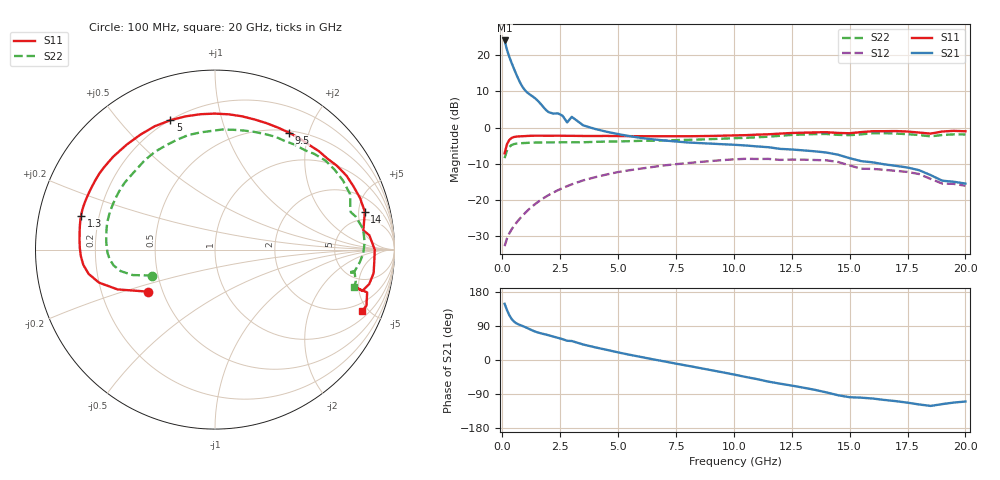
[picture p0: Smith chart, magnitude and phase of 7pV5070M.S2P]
! Infineon Technologies  Discrete & RF Semiconductors
! bfp620
! VCE = 0.50 V,  IC =  70 mA
! Common Emitter S-Parameters:  Sep 2002
# GHz  S  MA  R  50
!  f  S11  S21  S12  S22
! GHz  MAG  ANG  MAG  ANG  MAG  ANG  MAG  ANG
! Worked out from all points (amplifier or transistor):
!   59 points, 100 MHz to 20 GHz, reference 50 ohm
!   highest |S21| = 24.1 dB at 100 MHz (marker M1)
!   |S21| within 3 dB of that: start of sweep to 223.3 MHz
!   unconditionally stable (mu >= 1): start of sweep to 273.5 MHz; 598.9 MHz to 13.05 GHz; 14.34 GHz to end of sweep
!   at 1 GHz: K = 1.13, MAG = 14.6 dB, |S12| = -23.5 dB
!   at 5.5 GHz: K = 1.21, MAG = 1.9 dB, |S12| = -11.8 dB
!   at 20 GHz: K = 2.15, MAG = -5.8 dB, |S12| = -16.1 dB
!   S11 on the Smith chart (normalised r, x): 100 MHz: 0.42, -0.24; 1.3 GHz: 0.13, +0.12; 5 GHz: 0.20, +0.69; 9.5 GHz: 0.53, +1.69; 14 GHz: 3.60, +5.87; 20 GHz: 1.42, -4.56
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0.1  0.4389 -147.7  15.98 148.4  0.0229 27.2  0.3771 -157.5
0.2  0.5868 -157.8  11.93 132.1  0.0291 33.1  0.4798 -162.8
0.3  0.6719 -164.1  9.518 118.5  0.0343 37.2  0.5395 -167.2
0.4  0.7169 -169.1  7.853 108.5  0.039 40.5  0.5724 -171.2
0.5  0.7387 -173.4  6.545 101.6  0.0435 43.1  0.5898 -174.9
0.6  0.7486 -177.3  5.48 97.1  0.0479 45.2  0.5988 -178.2
0.8  0.7562 176.4  3.997 91.6  0.057 48.2  0.6069 176.2
1  0.762 171.6  3.224 86.5  0.0666 49.8  0.6117 171.9
1.3  0.7699 165.9  2.706 78.0  0.0816 50.3  0.6177 166.8
2  0.7701 152.9  1.631 65.3  0.1164 47.2  0.6227 155.1
2.6  0.7699 143.7  1.46 55.0  0.1454 42.1  0.6255 146.5
2.8  0.7677 140.2  1.177 50.8  0.1546 40.1  0.6263 143.3
3  0.7678 137.6  1.405 50.1  0.164 38.1  0.6251 141.0
3.5  0.7643 130.0  1.07 40.8  0.1862 32.7  0.6257 134.2
5  0.7624 109.0  0.812 20.1  0.2424 16.5  0.6418 114.9
7  0.7577 84.0  0.662 -3.7  0.2996 -4.6  0.6614 91.8
9.5  0.7711 57.7  0.588 -32.3  0.354 -31.6  0.7013 66.6
10.5  0.7843 48.1  0.565 -44.6  0.3691 -44.0  0.7195 57.2
13.5  0.8577 19.6  0.469 -78.7  0.3556 -77.6  0.8105 28.3
14  0.861 14.2  0.451 -85.5  0.3522 -84.4  0.8136 22.2
17  0.8934 -8.4  0.295 -108.6  0.2518 -108.1  0.8262 -1.5
20  0.8869 -22.7  0.168 -109.6  0.1568 -120.0  0.8022 -15.0
